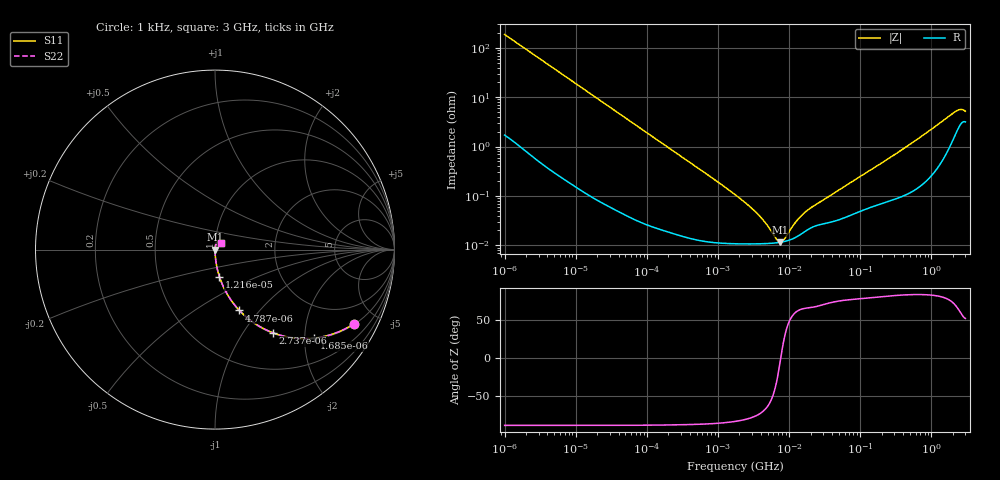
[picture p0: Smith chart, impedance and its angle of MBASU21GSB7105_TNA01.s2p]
! MBASU21GSB7105_TNA01  S-PARAMETER MODEL  ( Standard Model )
! Model Generated by TAIYO YUDEN Corporation (http://www.ty-top.com)
! Version 1.0
! TAIYO YUDEN Control No. 220601
! Copyright(c) 2013 TAIYO YUDEN CO.,LTD. All Rights Reserved.
! Product Description (link to TY-COMPAS)
! https://ds.yuden.co.jp/TYCOMPAS/or/detail?pn=MBASU21GSB7105KTNA01&u=M
! Products Name : Multilayer Ceramic Capacitors
! Characteristics :
!  Capacitance : 1 [uF] , Rated Voltage : 50 [V] , TCC : X7R
!  Case Size : 2.0 x 1.25 / 0.079 x 0.049 [mm/inch] , Thickness : 1.25 / 0.049 [mm/inch]
!  (Conditions: Temperature = 25 [degC] , DC Bias Voltage = 0 [V])
! External Node Assignments :
!  1  o---| |---o  2
! GND o---------o GND
! Frequency Range : 1kHz  -  3GHz  [ 401 STEP ]
# MHZ S RI R 50
! Freq[MHz].  S11 Real  S11 Imag  S21 Real  S21 Imag  S12 Real  S12 Imag  S22 Real  S22 Imag
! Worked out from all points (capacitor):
!   401 points, 1 kHz to 3 GHz, reference 50 ohm
!   read as one part in series: C = 850 nF near 1.077 kHz
!   lowest |Z| = 11.5 mohm at 7.414 MHz (marker M1)
!   series resonance near 7.614 MHz, so ESL is about 510 pH
!   S11 on the Smith chart (normalised r, x): 1 kHz: 1.03, -3.74; 1.685 kHz: 1.02, -2.23; 2.737 kHz: 1.01, -1.37; 4.787 kHz: 1.01, -0.79; 12.16 kHz: 1.00, -0.31; 3 GHz: 1.06, +0.08
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0.001  0.7754 -0.4128  0.2246 0.4128  0.2246 0.4128  0.7754 -0.4128
0.001685  0.5529 -0.4928  0.4471 0.4928  0.4471 0.4928  0.5529 -0.4928
0.002737  0.3222 -0.4633  0.6778 0.4633  0.6778 0.4633  0.3222 -0.4633
0.004787  0.1362 -0.3391  0.8638 0.3391  0.8638 0.3391  0.1362 -0.3391
0.007215  0.0658 -0.2441  0.9342 0.2441  0.9342 0.2441  0.0658 -0.2441
0.01216  0.0248 -0.1516  0.9752 0.1516  0.9752 0.1516  0.0248 -0.1516
0.033275  0.0038 -0.0569  0.9962 0.0569  0.9962 0.0569  0.0038 -0.0569
0.147855  0.00038 -0.013  0.9996 0.013  0.9996 0.013  0.00038 -0.013
1.732051  0.000108 -0.00106  0.9999 0.00106  0.9999 0.00106  0.000108 -0.00106
3.651041  0.000107 -0.00041  0.9999 0.00041  0.9999 0.00041  0.000107 -0.00041
4.739869  0.000108 -0.000252  0.9999 0.000252  0.9999 0.000252  0.000108 -0.000252
6.629817  0.000112 -7.12e-05  0.9999 7.12e-05  0.9999 7.12e-05  0.000112 -7.12e-05
7.414467  0.000115 -1.36e-05  0.9999 1.36e-05  0.9999 1.36e-05  0.000115 -1.36e-05
7.988506  0.000117 2.48e-05  0.9999 -2.48e-05  0.9999 -2.48e-05  0.000117 2.48e-05
8.606987  0.000119 6.34e-05  0.9999 -6.34e-05  0.9999 -6.34e-05  0.000119 6.34e-05
11.59828  0.000138 0.000223  0.9999 -0.000223  0.9999 -0.000223  0.000138 0.000223
13.97519  0.000161 0.000327  0.9998 -0.000327  0.9998 -0.000327  0.000161 0.000327
21.06097  0.000232 0.000553  0.9998 -0.000553  0.9998 -0.000553  0.000232 0.000553
256.0921  0.000818 0.00579  0.9992 -0.00579  0.9992 -0.00579  0.000818 0.00579
2144.796  0.0188 0.0463  0.9812 -0.0463  0.9812 -0.0463  0.0188 0.0463
2489.759  0.0279 0.0471  0.9721 -0.0471  0.9721 -0.0471  0.0279 0.0471
3000  0.0322 0.0387  0.9678 -0.0387  0.9678 -0.0387  0.0322 0.0387
